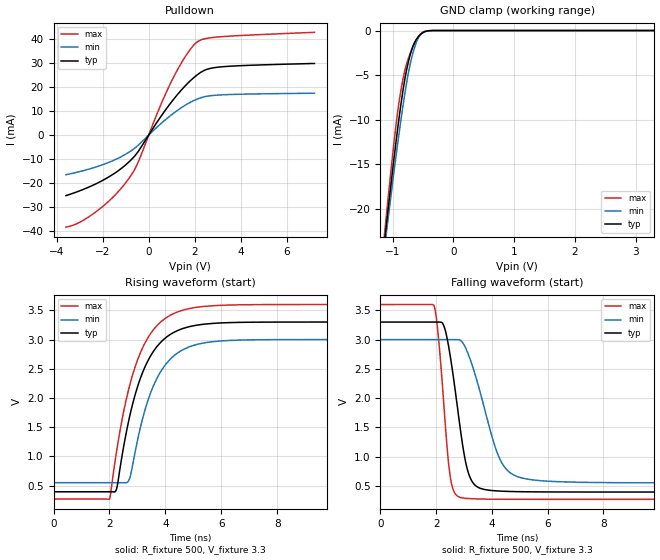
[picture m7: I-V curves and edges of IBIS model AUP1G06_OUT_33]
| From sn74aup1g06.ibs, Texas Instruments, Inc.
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[Model]   AUP1G06_OUT_33
Model_type  Open_drain
Enable   Active-Low
Vref =   3.3
Rref =   1E6
Cref =   30p
Vmeas =   1.65
| variable   typ   min   max
C_comp   1.56pF   1.29pF   1.96pF
| C_pulldown   1.90pF   1.64pF   2.45pF
| C_tri-state   1.56pF   1.29pF   1.96pF
[Temperature Range]   40   100   -40
| Ambient temperature   25   85   -40
[Voltage range]   3.3   3   3.6
[Pullup Reference]   3.3   3.3   3.3
[POWER Clamp Reference]   3.3   3.3   3.3
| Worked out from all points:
|   slope of the pulldown table from 0 to 0.495 V, typ, clamps not added: 68.4 ohm
|   GND clamp passes 1 mA (typ) near -0.61 V on its own axis
|   rising waveform, R_fixture 500, V_fixture 3.3: 20-80 % time 1.03ns typ, 1.01ns min, 1.06ns max; typ from 0.394 V to 3.3 V
|   falling waveform, R_fixture 500, V_fixture 3.3: 20-80 % time 524ps typ, 886ps min, 333ps max; typ from 3.3 V to 0.394 V
[GND Clamp]
| AUP1G06_OUT_33
|   Voltage   I(typ)   I(min)   I(max)
-3.6V     -193.5mA   -179.7mA   -210.2mA
-1.125V   -23.21mA   -23.99mA   -22.31mA
-1.1V     -21.68mA   -22.59mA   -20.6mA
-1.075V   -20.16mA   -21.19mA   -18.91mA
-940mV    -12.31mA   -13.93mA   -10.42mA
-885mV    -9.391mA   -11.14mA   -7.65mA
-820mV    -6.351mA   -8.054mA   -5.152mA
-740mV    -3.533mA   -4.796mA   -3.135mA
-655mV    -1.602mA   -2.299mA   -1.69mA
-580mV    -733.4uA   -904.6uA   -734uA
-495mV    -220.6uA   -214.9uA   -155.7uA
3.3V      255.6pA    757pA      63.57pA
[Pulldown]
| AUP1G06_OUT_33
|   Voltage   I(typ)   I(min)   I(max)
-3.6V     -25.22mA   -16.54mA   -38.34mA
-2.98V    -23.15mA   -15.18mA   -36.21mA
-2.195V   -19.84mA   -13mA      -31.21mA
-1.455V   -15.73mA   -10.24mA   -24.88mA
-855mV    -11.15mA   -7.128mA   -17.97mA
-490mV    -7.269mA   -4.538mA   -11.95mA
415mV     6.109mA    3.748mA    10.09mA
1.015V    14.06mA    8.579mA    22.82mA
1.6V      20.58mA    12.45mA    32.78mA
2.085V    24.83mA    14.83mA    38.52mA
3.09V     28.26mA    16.63mA    40.81mA
7.2V      29.73mA    17.36mA    42.67mA
[Ramp]
| AUP1G06_OUT_33
| variable   typ   min   max
dV/dt_r   1.74/1.03E-09   1.47/1.01E-09   2.00/1.06E-09
dV/dt_f   1.74/5.24E-10   1.47/8.88E-10   2.00/3.35E-10
R_load = 500
[Rising Waveform]
| AUP1G06_OUT_33
R_fixture =   500
C_fixture =   0
L_fixture =   0
V_fixture =   3.3
V_fixture_min = 3
V_fixture_max = 3.6
|   Time   V(typ)   V(min)   V(max)
0s        394.1mV    550mV      269.3mV
1.995ns   394.1mV    550.1mV    266.1mV
2.255ns   443.2mV    550.1mV    1.084V
2.685ns   1.599V     582.9mV    2.142V
3.09ns    2.313V     1.458V     2.754V
3.42ns    2.676V     2.016V     3.063V
3.795ns   2.933V     2.42V      3.283V
4.8ns     3.213V     2.864V     3.524V
7.275ns   3.298V     2.996V     3.598V
30.7ns    3.3V       3V         3.6V
[Falling Waveform]
| AUP1G06_OUT_33
R_fixture =   500
C_fixture =   0
L_fixture =   0
V_fixture =   3.3
V_fixture_min = 3
V_fixture_max = 3.6
|   Time   V(typ)   V(min)   V(max)
0s        3.3V       3V         3.6V
1.925ns   3.3V       3V         3.579V
2.255ns   3.259V     3V         2.03V
2.495ns   2.752V     3V         694.7mV
2.9ns     1.364V     2.975V     297mV
3.13ns    765.9mV    2.779V     283.7mV
3.405ns   507.5mV    2.393V     277.2mV
4.3ns     410.1mV    946.6mV    270.6mV
5.23ns    398.5mV    618.5mV    269.5mV
30.7ns    394.1mV    550mV      269.3mV
